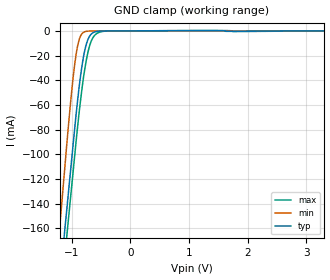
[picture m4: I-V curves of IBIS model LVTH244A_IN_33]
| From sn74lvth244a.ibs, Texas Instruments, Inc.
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[Model]   LVTH244A_IN_33
Model_type  Input
Vinl=0.8
Vinh=2.0
| variable   typ   min   max
C_comp   3.84pF   3.07pF   5.22pF
[Temperature Range]   40   -40   100
| Ambient temperature   25   -40   85
[Voltage range]   3.3   3   3.6
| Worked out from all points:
|   GND clamp passes 1 mA (typ) near -0.62 V on its own axis
[GND Clamp]
| LVTH244A_IN_33
|   Voltage   I(typ)   I(min)   I(max)
-5.5V     -2.408A    -2.647A    -2.409A
-1.22V    -209.4mA   -166.1mA   -230.4mA
-1.125V   -163.2mA   -113.2mA   -184.6mA
-1.075V   -138.9mA   -85.42mA   -160.5mA
-975mV    -90.33mA   -36.31mA   -112.3mA
-900mV    -55.43mA   -11.64mA   -76.74mA
-825mV    -27.57mA   -2.158mA   -45.91mA
-775mV    -14.79mA   -631.5uA   -29.62mA
-725mV    -6.832mA   -223.9uA   -17.14mA
-650mV    -1.834mA   -140.7uA   -6.297mA
-405mV    -96.3uA    -83.61uA   -155.7uA
3.3V      19.45pA    12.56pA    -1.138uA
